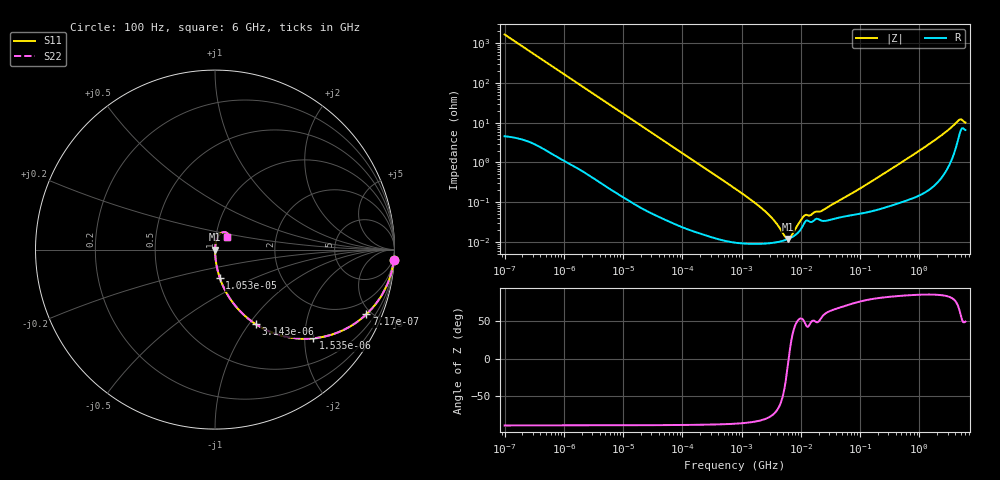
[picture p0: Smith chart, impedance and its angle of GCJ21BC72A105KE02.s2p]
!Murata Part Number: GCJ21BC72A105KE02
!These Parameters are Measured in Series Mode Connection
!Data Generated on Mar 13, 2026
!  o--ll--o
!Port1  Port2
!  o------o
!Operation Temp=25[degC], DC Bias Voltage=0[V]
!Freq. Start=100[Hz] Stop=6[GHz] 401[Steps]
# Hz S RI R 50
!Freq.(Hz) S11(Real) S11(Imag) S21(Real) S21(Imag) S12(Real) S12(Imag) S22(Real) S22(Imag)
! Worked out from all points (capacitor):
!   401 points, 100 Hz to 6 GHz, reference 50 ohm
!   read as one part in series: C = 954 nF near 109 Hz
!   lowest |Z| = 11.9 mohm at 6.075 MHz (marker M1)
!   series resonance near 6.241 MHz, so ESL is about 680 pH
!   S11 on the Smith chart (normalised r, x): 100 Hz: 1, -33; 717 Hz: 1.03, -4.68; 1.535 kHz: 1.02, -2.19; 3.143 kHz: 1.01, -1.07; 10.53 kHz: 1.00, -0.32; 6 GHz: 1.13, +0.15
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100  0.9962 -0.0598  0.00375 0.0598  0.00375 0.0598  0.9962 -0.0598
335  0.9604 -0.1922  0.0396 0.1922  0.0396 0.1922  0.9604 -0.1922
717  0.8439 -0.3598  0.1561 0.3598  0.1561 0.3598  0.8439 -0.3598
1535  0.5454 -0.4944  0.4546 0.4944  0.4546 0.4944  0.5454 -0.4944
2008  0.4138 -0.4888  0.5862 0.4888  0.5862 0.4888  0.4138 -0.4888
3143  0.2258 -0.4144  0.7742 0.4144  0.7742 0.4144  0.2258 -0.4144
5378  0.0919 -0.2852  0.9081 0.2852  0.9081 0.2852  0.0919 -0.2852
10527  0.0265 -0.1569  0.9735 0.1569  0.9735 0.1569  0.0265 -0.1569
40335  0.00221 -0.0423  0.9978 0.0423  0.9978 0.0423  0.00221 -0.0423
774597  0.000101 -0.00221  0.9999 0.00221  0.9999 0.00221  0.000101 -0.00221
2594782  9.16e-05 -0.000556  0.9999 0.000556  0.9999 0.000556  9.16e-05 -0.000556
3712478  9.72e-05 -0.000304  0.9999 0.000304  0.9999 0.000304  9.72e-05 -0.000304
5311619  0.00011 -9.09e-05  0.9999 9.09e-05  0.9999 9.09e-05  0.00011 -9.09e-05
6075234  0.000118 -1.51e-05  0.9999 1.51e-05  0.9999 1.51e-05  0.000118 -1.51e-05
6948629  0.00013 6.11e-05  0.9999 -6.11e-05  0.9999 -6.11e-05  0.00013 6.11e-05
1.087309e7  0.000257 0.000334  0.9997 -0.000334  0.9997 -0.000334  0.000257 0.000334
1.555665e7  0.000321 0.000389  0.9997 -0.000389  0.9997 -0.000389  0.000321 0.000389
2.434276e7  0.000338 0.000552  0.9997 -0.000552  0.9997 -0.000552  0.000338 0.000552
3.124326e8  0.000833 0.00637  0.9992 -0.00637  0.9992 -0.00637  0.000833 0.00637
1.791126e9  0.00386 0.0355  0.9961 -0.0355  0.9961 -0.0355  0.00386 0.0355
4.586474e9  0.0493 0.0977  0.9507 -0.0977  0.9507 -0.0977  0.0493 0.0977
6e9  0.0665 0.0677  0.9335 -0.0677  0.9335 -0.0677  0.0665 0.0677
